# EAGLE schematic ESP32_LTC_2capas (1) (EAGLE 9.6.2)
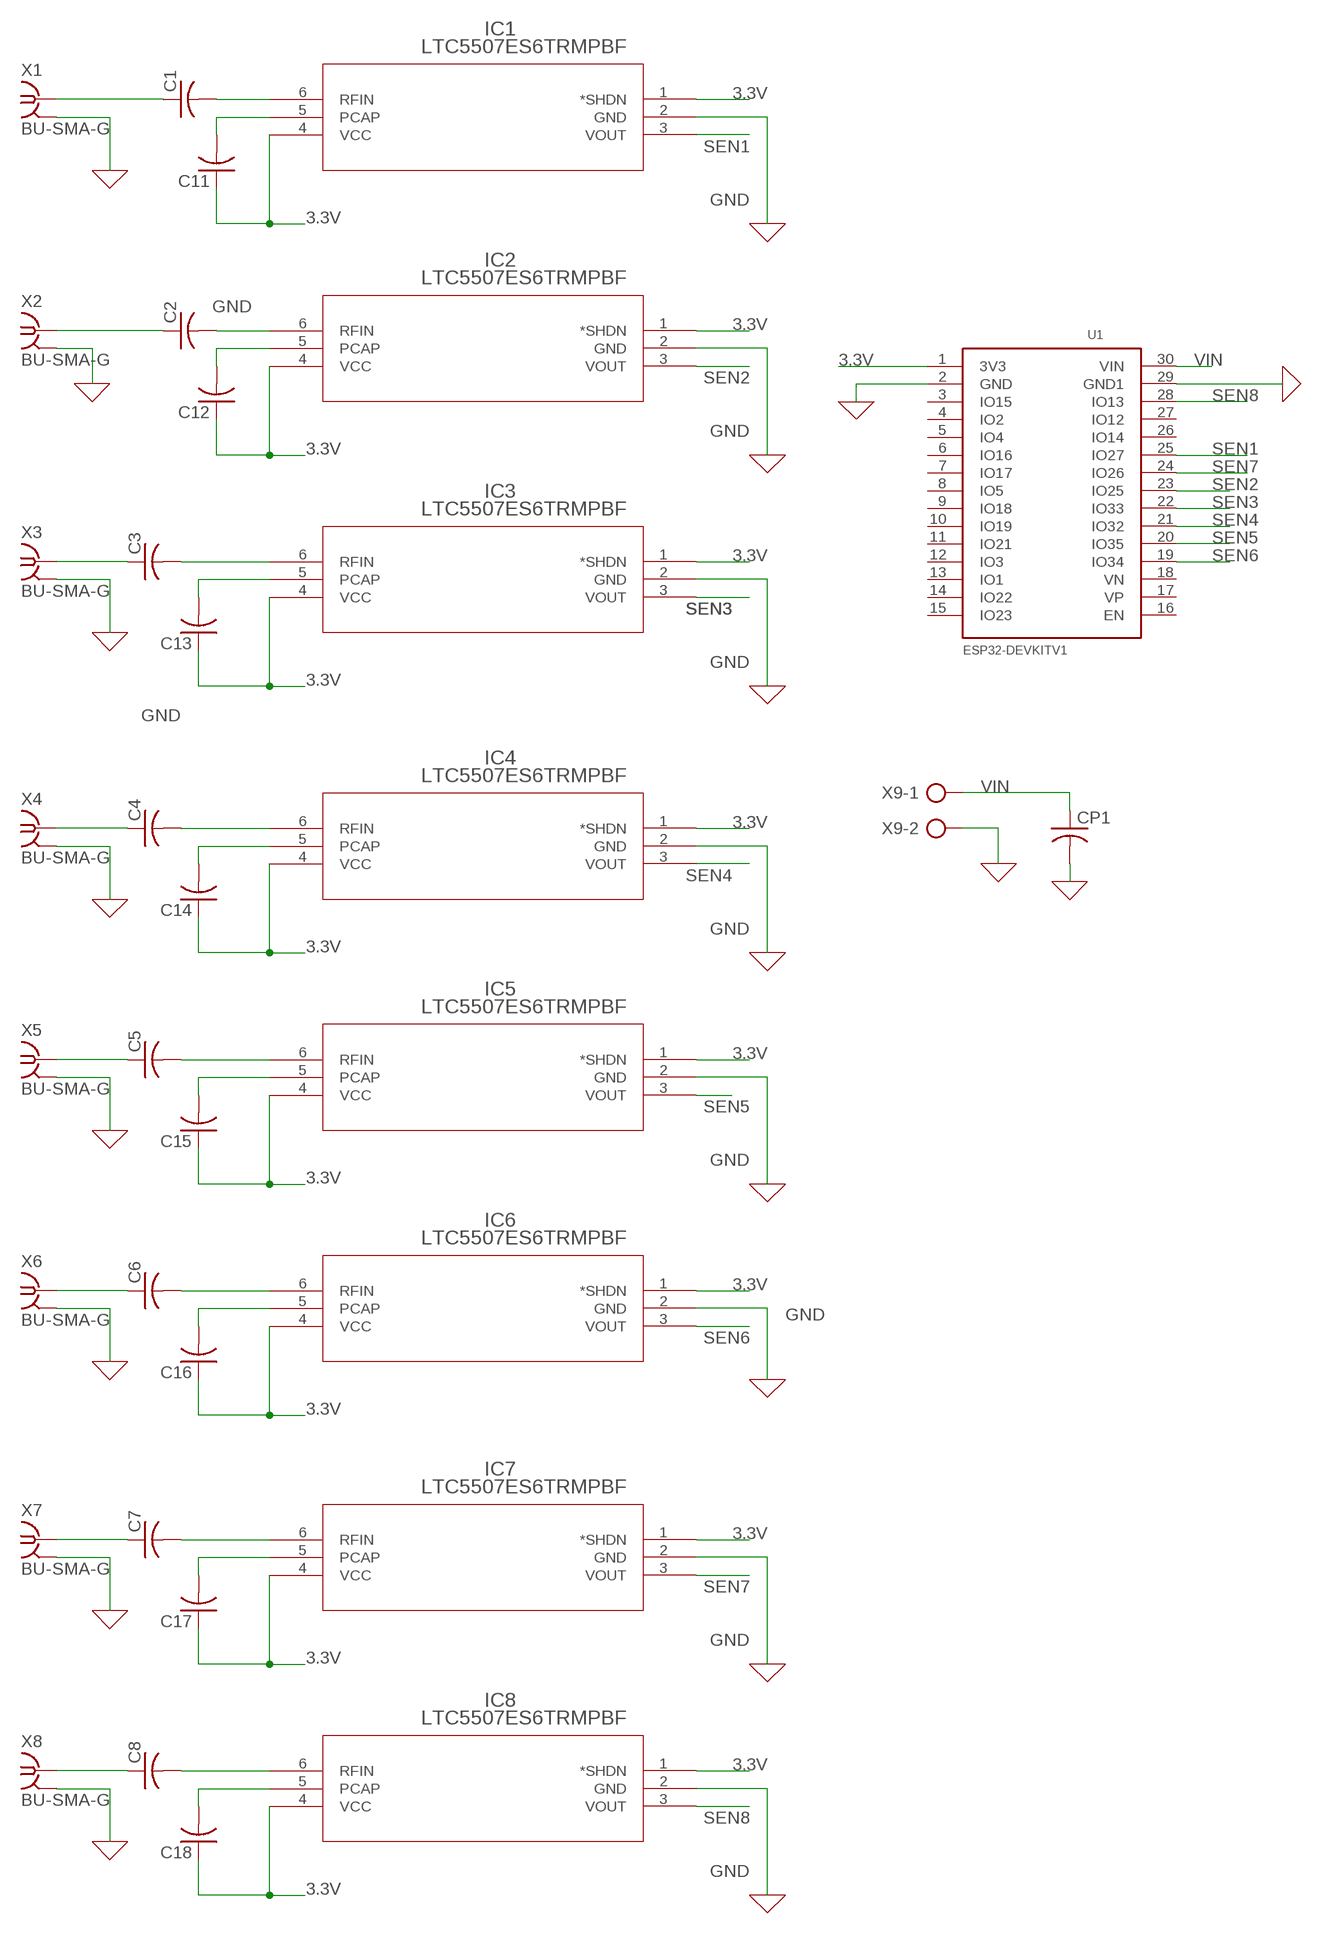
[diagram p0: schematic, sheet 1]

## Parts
C1  RCL_C-USC0805  [RCL_C0805]
C2  RCL_C-USC0805  [RCL_C0805]
C3  RCL_C-USC0805  [RCL_C0805]
C4  RCL_C-USC0805  [RCL_C0805]
C5  RCL_C-USC0805  [RCL_C0805]
C6  RCL_C-USC0805  [RCL_C0805]
C7  RCL_C-USC0805  [RCL_C0805]
C8  RCL_C-USC0805  [RCL_C0805]
C11  RCL_C-USC0805  [RCL_C0805]
C12  RCL_C-USC0805  [RCL_C0805]
C13  RCL_C-USC0805  [RCL_C0805]
C14  RCL_C-USC0805  [RCL_C0805]
C15  RCL_C-USC0805  [RCL_C0805]
C16  RCL_C-USC0805  [RCL_C0805]
C17  RCL_C-USC0805  [RCL_C0805]
C18  RCL_C-USC0805  [RCL_C0805]
CP1  RCL_C-USC0805  [RCL_C0805]
IC1  LTC5507ES6TRMPBF  [SOT-23_S6]
IC2  LTC5507ES6TRMPBF  [SOT-23_S6]
IC3  LTC5507ES6TRMPBF  [SOT-23_S6]
IC4  LTC5507ES6TRMPBF  [SOT-23_S6]
IC5  LTC5507ES6TRMPBF  [SOT-23_S6]
IC6  LTC5507ES6TRMPBF  [SOT-23_S6]
IC7  LTC5507ES6TRMPBF  [SOT-23_S6]
IC8  LTC5507ES6TRMPBF  [SOT-23_S6]
U1  ESP32-DEVKITV1_ESP32DEVKITV1  [ESP32-DEVKITV1_ESP32-DEVKITV1]
X1  BU-SMA-G  [BU-SMA-G]
X2  BU-SMA-G  [BU-SMA-G]
X3  BU-SMA-G  [BU-SMA-G]
X4  BU-SMA-G  [BU-SMA-G]
X5  BU-SMA-G  [BU-SMA-G]
X6  BU-SMA-G  [BU-SMA-G]
X7  BU-SMA-G  [BU-SMA-G]
X8  BU-SMA-G  [BU-SMA-G]
X9  CGS_02_AK500/2  [CGS_02_AK500/2]

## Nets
3.3V: C11.1 C12.1 C13.1 C14.1 C15.1 C16.1 C17.1 C18.1 IC1.1(*SHDN) IC1.4(VCC) IC2.1(*SHDN) IC2.4(VCC) IC3.1(*SHDN) IC3.4(VCC) IC4.1(*SHDN) IC4.4(VCC) IC5.1(*SHDN) IC5.4(VCC) IC6.1(*SHDN) IC6.4(VCC) IC7.1(*SHDN) IC7.4(VCC) IC8.1(*SHDN) IC8.4(VCC) U1.1(3V3)
GND: CP1.2 IC1.2(GND) IC2.2(GND) IC3.2(GND) IC4.2(GND) IC5.2(GND) IC6.2(GND) IC7.2(GND) IC8.2(GND) U1.2(GND) U1.29(GND1) X1.2 X1.3 X1.4 X1.5 X2.2 X2.3 X2.4 X2.5 X3.2 X3.3 X3.4 X3.5 X4.2 X4.3 X4.4 X4.5 X5.2 X5.3 X5.4 X5.5 X6.2 X6.3 X6.4 X6.5 X7.2 X7.3 X7.4 X7.5 X8.2 X8.3 X8.4 X8.5 X9.2
N$1: C11.2 IC1.5(PCAP)
N$2: C1.2 IC1.6(RFIN)
N$3: C1.1 X1.1
N$4: C12.2 IC2.5(PCAP)
N$5: C2.2 IC2.6(RFIN)
N$6: C2.1 X2.1
N$7: C13.2 IC3.5(PCAP)
N$8: C3.2 IC3.6(RFIN)
N$9: C3.1 X3.1
N$10: C14.2 IC4.5(PCAP)
N$11: C4.2 IC4.6(RFIN)
N$12: C4.1 X4.1
N$13: C15.2 IC5.5(PCAP)
N$14: C5.2 IC5.6(RFIN)
N$15: C5.1 X5.1
N$16: C16.2 IC6.5(PCAP)
N$17: C6.2 IC6.6(RFIN)
N$18: C6.1 X6.1
N$19: C17.2 IC7.5(PCAP)
N$20: C7.2 IC7.6(RFIN)
N$21: C7.1 X7.1
N$22: C18.2 IC8.5(PCAP)
N$23: C8.2 IC8.6(RFIN)
N$24: C8.1 X8.1
SEN1: IC1.3(VOUT) U1.25(IO27)
SEN2: IC2.3(VOUT) U1.23(IO25)
SEN3: IC3.3(VOUT) U1.22(IO33)
SEN4: IC4.3(VOUT) U1.21(IO32)
SEN5: IC5.3(VOUT) U1.20(IO35)
SEN6: IC6.3(VOUT) U1.19(IO34)
SEN7: IC7.3(VOUT) U1.24(IO26)
SEN8: IC8.3(VOUT) U1.28(IO13)
VIN: CP1.1 U1.30(VIN) X9.1
Unconnected: U1.3(IO15) U1.4(IO2) U1.5(IO4) U1.6(IO16) U1.7(IO17) U1.8(IO5) U1.9(IO18) U1.10(IO19) U1.11(IO21) U1.12(IO3) U1.13(IO1) U1.14(IO22) U1.15(IO23) U1.16(EN) U1.17(VP) U1.18(VN) U1.26(IO14) U1.27(IO12)

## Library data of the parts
C1-C8 C11-C18 CP1 = RDS_SasPe:RCL_C-US: CAPACITOR, American symbol; SPICEPREFIX: C
IC1-IC8 = LTC5507ES6TRMPBF:LTC5507ES6TRMPBF: Check availability; AVAILABILITY: In Stock; CHECK_PRICES: https://www.snapeda.com/parts/LTC5507ES6%23TRMPBF/Analog+Devices/view-part/?ref=eda; DESCRIPTION: 100kHz to 1GHz RF Power Detector; MF: Analog Devices; MP: LTC5507ES6#TRMPBF; PACKAGE: SOT-6 Analog Devices; PRICE: None; PURCHASE-URL: https://www.snapeda.com/api/url_track_click_mouser/?unipart_id=4331394&manufacturer=Analog Devices&part_name=LTC5507ES6#TRMPBF&search_term=None; SNAPEDA_LINK: https://www.snapeda.com/parts/LTC5507ES6%23TRMPBF/Analog+Devices/view-part/?ref=snap
U1 = RDS_SasPe:ESP32-DEVKITV1_ESP32DEVKITV1
X1-X8 = con-coax:BU-SMA-G: FEMALE SMA CONNECTOR; OC_FARNELL: unknown; OC_NEWARK: unknown
X9 = CR30_2020_C:CGS_02_AK500/2: CONNECTOR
